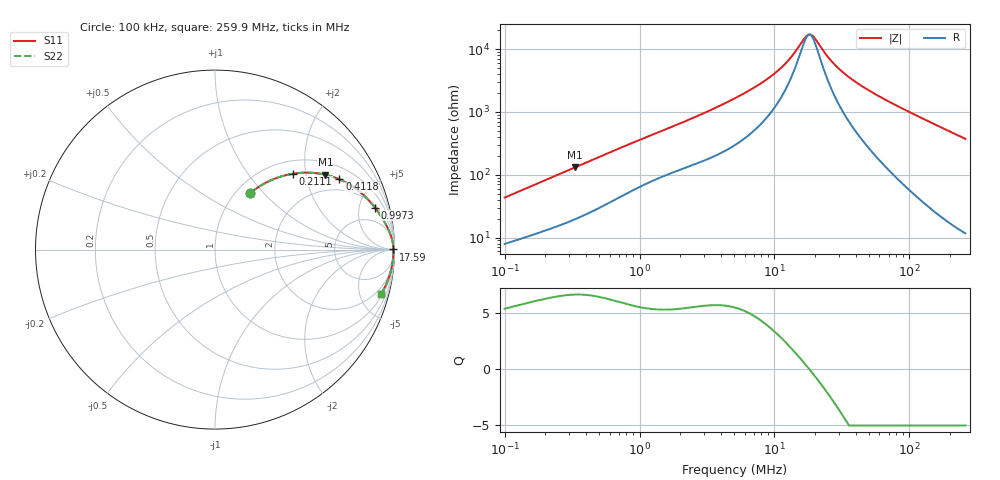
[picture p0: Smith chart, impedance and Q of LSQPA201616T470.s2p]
! LSQPA201616T470  S-PARAMETER MODEL  ( General Type )
! Model Generated by TAIYO YUDEN Corporation (http://www.ty-top.com)
! Version 2.0
! TAIYO YUDEN Control No. 100810NF25SB-FKC
! Copyright(c) 2007 TAIYO YUDEN CO.,LTD. All Rights Reserved.
! Product Description (link to TY-COMPAS)
! https://ds.yuden.co.jp/TYCOMPAS/or/detail?pn=LSQPA201616T470K&u=M
! Products Name : Inductors
! Characteristics :
!  Inductance : 47 uH , SRF(min) : 11 MHz , DC Resistance(max) : 5.59 Ohm
!  Rated Current : Saturation :150 mA , Temp Rise : 150 mA (40 degC)
!  Case Size : 2.0 x 1.6 / 0.079 x 0.063 [mm/inch] , Thickness : 1.6 / 0.063 [mm/inch]
!  (Conditions: Temperature = 25 degC , DC Bias Current/Voltage = 0A / 0V)
! External Node Assignments :
!  1  o---GGG---o  2
! GND o---------o GND
! Frequency Range : 0.1MHz  -  259.929867MHz  [ 402 STEP ]
# MHz S RI R 50
! Freq[MHz].  S11 Real  S11 Imag  S21 Real  S21 Imag  S12 Real  S12 Imag  S22 Real  S22 Imag
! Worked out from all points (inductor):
!   401 points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, 100 kHz to 259.9 MHz, reference 50 ohm
!   read as one part in series: L = 66.4 uH near 104 kHz
!   highest Q = 6.64 at 331.7 kHz (marker M1), where L = 62.1 uH
!   self-resonance near 17.94 MHz
!   S11 on the Smith chart (normalised r, x): 100 kHz: 1.16, +0.85; 211.1 kHz: 1.27, +1.70; 411.8 kHz: 1.48, +3.16; 997.3 kHz: 2.27, +7.03; 17.59 MHz: open; 259.9 MHz: 1.23, -7.46
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0.1  0.1976 0.3159  0.8024 -0.3159  0.8024 -0.3159  0.1976 0.3159
0.211063  0.4348 0.4229  0.5652 -0.4229  0.5652 -0.4229  0.4348 0.4229
0.331715  0.6146 0.4172  0.3854 -0.4172  0.3854 -0.4172  0.6146 0.4172
0.37324  0.6587 0.4048  0.3413 -0.4048  0.3413 -0.4048  0.6587 0.4048
0.411788  0.6932 0.3916  0.3068 -0.3916  0.3068 -0.3916  0.6932 0.3916
0.622234  0.8101 0.3194  0.1899 -0.3194  0.1899 -0.3194  0.8101 0.3194
0.997345  0.8913 0.2337  0.1087 -0.2337  0.1087 -0.2337  0.8913 0.2337
1.393082  0.9265 0.1833  0.0735 -0.1833  0.0735 -0.1833  0.9265 0.1833
2.826922  0.97 0.1034  0.03 -0.1034  0.03 -0.1034  0.97 0.1034
5.098332  0.9859 0.0579  0.0141 -0.0579  0.0141 -0.0579  0.9859 0.0579
7.703854  0.9908 0.0349  0.00917 -0.0349  0.00917 -0.0349  0.9908 0.0349
10.55121  0.9928 0.0208  0.00721 -0.0208  0.00721 -0.0208  0.9928 0.0208
13.09818  0.9936 0.0122  0.00642 -0.0122  0.00642 -0.0122  0.9936 0.0122
16.58275  0.9941 0.00332  0.00591 -0.00332  0.00591 -0.00332  0.9941 0.00332
17.59008  0.9942 0.00114  0.00583 -0.00114  0.00583 -0.00114  0.9942 0.00114
19.02902  0.9943 -0.00177  0.00575 0.00177  0.00575 0.00177  0.9943 -0.00177
25.55487  0.9943 -0.013  0.0057 0.013  0.0057 0.013  0.9943 -0.013
32.35335  0.994 -0.0227  0.00596 0.0227  0.00596 0.0227  0.994 -0.0227
45.19087  0.9931 -0.0388  0.00691 0.0388  0.00691 0.0388  0.9931 -0.0388
71.02397  0.9899 -0.0677  0.0101 0.0677  0.0101 0.0677  0.9899 -0.0677
138.5695  0.9747 -0.1367  0.0253 0.1367  0.0253 0.1367  0.9747 -0.1367
259.9299  0.9263 -0.2462  0.0737 0.2462  0.0737 0.2462  0.9263 -0.2462
